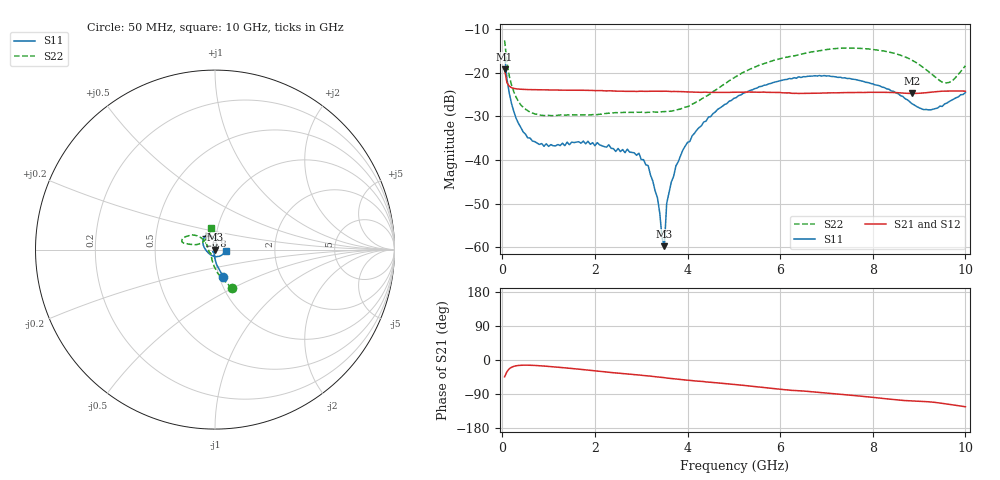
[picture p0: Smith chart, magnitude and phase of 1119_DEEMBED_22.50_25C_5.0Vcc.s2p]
!Hittite Microwave Corp.
!Digital Attenuator/PhaseShifter Rev 1.4.0
!Filename: C:\DATA\DATA\1119_DEEMBED_22.50_25C_5.0Vcc.s2p
!VNA ID: Agilent Technologies,N5224A,MY51441122,A.10.45.03
!Device type:
!2 Port Calibration.
!Temp(C): 25
!Lot Number:
!Serial Number:
!Operator:
!Misc:
!Attenuator:  22.500
# GHZ S DB R 50.0
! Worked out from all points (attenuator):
!   200 points, 50 MHz to 10 GHz, reference 50 ohm
!   highest |S21| = -19.24 dB at 50 MHz (marker M1); lowest = -24.8 dB at 8.85 GHz (marker M2)
!   lowest |S11| = -59.8 dB at 3.5 GHz (marker M3), VSWR 1.00, Z = 50.1 + j0.0318 ohm
!   |S11| at or under -10 dB: start of sweep to end of sweep
!   |S22| runs from -29.8 to -12.6 dB; largest |S21 - S12| = 0.00017
!   S11 on the Smith chart (normalised r, x): 50 MHz: 1.05, -0.33; 6.8 GHz: 0.89, +0.14; 10 GHz: 1.13, -0.01
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0.05  -15.89 -73.0  -19.24 -44.4  -19.25 -44.5  -12.60 -66.6
0.1  -21.38 -83.5  -22.25 -30.9  -22.24 -30.9  -17.56 -83.5
0.2  -27.09 -92.4  -23.43 -19.1  -23.43 -19.1  -22.83 -100.1
0.55  -34.94 -109.0  -23.86 -13.6  -23.85 -13.6  -28.71 -125.8
0.9  -36.86 -117.6  -23.92 -16.0  -23.92 -16.0  -29.81 -135.1
1.75  -35.67 -126.4  -24.02 -25.4  -24.03 -25.4  -29.67 -139.8
2.95  -38.44 -104.8  -24.25 -39.5  -24.26 -39.6  -29.07 -158.8
3.15  -41.29 -96.2  -24.25 -41.9  -24.26 -42.0  -29.06 -164.8
3.4  -52.14 -93.2  -24.25 -45.2  -24.26 -45.3  -29.00 -172.2
3.45  -57.84 -29.8  -24.25 -46.0  -24.26 -46.0  -28.94 -174.1
3.5  -59.76 18.0  -24.23 -46.6  -24.24 -46.6  -28.91 -175.7
3.55  -49.96 59.2  -24.24 -47.6  -24.26 -47.6  -28.90 -177.6
3.75  -41.32 69.3  -24.30 -50.0  -24.31 -50.1  -28.57 174.7
3.9  -37.71 67.1  -24.34 -52.0  -24.35 -52.0  -28.10 168.1
4.45  -30.19 74.6  -24.51 -58.5  -24.52 -58.5  -25.09 147.4
5.05  -25.72 87.7  -24.47 -64.9  -24.49 -65.0  -20.85 139.5
6.7  -20.77 121.0  -24.68 -83.9  -24.68 -83.9  -15.19 154.5
6.8  -20.76 123.0  -24.69 -85.0  -24.70 -85.0  -15.04 155.8
8.35  -23.80 165.1  -24.52 -103.0  -24.52 -103.0  -15.25 168.2
8.85  -27.13 -163.2  -24.76 -107.9  -24.75 -108.0  -17.15 167.9
9.55  -27.15 -60.1  -24.21 -115.4  -24.22 -115.4  -22.29 138.9
10  -24.55 -5.1  -24.23 -123.4  -24.24 -123.3  -18.40 99.6
